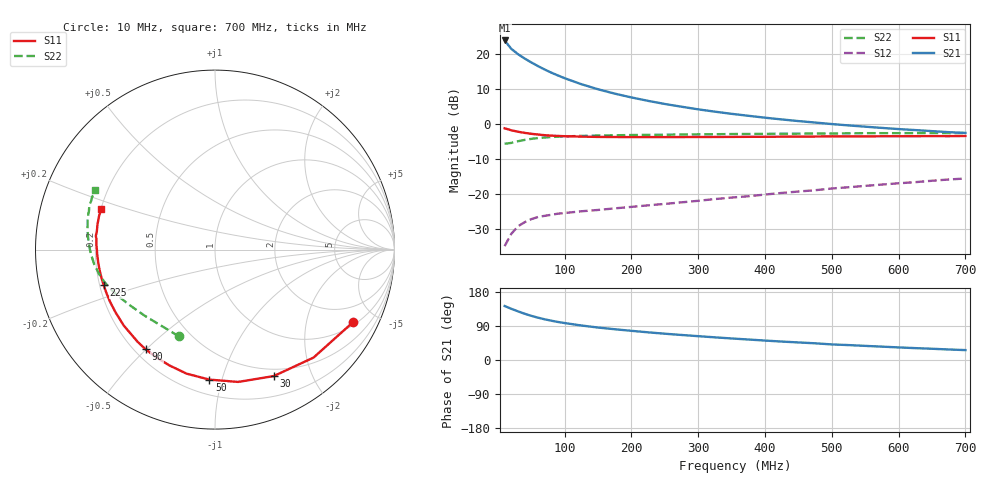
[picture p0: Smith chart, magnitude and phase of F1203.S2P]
! Date: Mon Aug 07 16:10:10 1995
# MHZ  S  MA  R  50.0000
!  POLYFET RF DEVICES
!  F1203
!  S PARAMETERS
!  VDS=12.5V, IDQ=200mA
! FREQ  S11MAG  S11ANG  S21MAG  S21ANG  S12MAG  S12ANG  S22MAG  S22ANG
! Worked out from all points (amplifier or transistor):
!   34 points, 10 MHz to 700 MHz, reference 50 ohm
!   highest |S21| = 23.8 dB at 10 MHz (marker M1)
!   |S21| within 3 dB of that: start of sweep to 24.06 MHz
!   unconditionally stable (mu >= 1): 188.4 MHz to end of sweep
!   at 60 MHz: K = 0.37, MSG = 21.5 dB, |S12| = -26.5 dB
!   at 300 MHz: K = 1.25, MAG = 10.0 dB, |S12| = -21.9 dB
!   at 700 MHz: K = 1.24, MAG = 3.5 dB, |S12| = -15.5 dB
!   S11 on the Smith chart (normalised r, x): 10 MHz: 1.14, -3.75; 30 MHz: 0.42, -1.49; 50 MHz: 0.30, -0.91; 90 MHz: 0.24, -0.50; 225 MHz: 0.22, -0.15; 700 MHz: 0.20, +0.17
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10  0.8697 -27.6  15.52 142.5  0.01819 56.1  0.5237 -112.5
20  0.8145 -47.6  11.79 135.1  0.02725 49.0  0.5383 -137.0
30  0.7771 -65.1  9.908 128.4  0.03489 44.9  0.5685 -147.3
40  0.7484 -80.1  8.584 122.1  0.03992 42.1  0.5939 -153.5
50  0.7251 -92.4  7.539 116.5  0.04413 39.8  0.6148 -157.9
60  0.7091 -102.8  6.689 111.7  0.0474 38.0  0.6308 -161.4
70  0.6935 -111.5  5.982 107.4  0.0492 35.8  0.6431 -164.0
80  0.6835 -118.7  5.391 103.7  0.05098 34.5  0.6521 -166.2
90  0.6769 -124.8  4.914 100.3  0.05283 34.7  0.6605 -168.1
100  0.6706 -130.0  4.495 97.5  0.054 34.0  0.6655 -169.8
125  0.6615 -140.3  3.693 91.1  0.05713 33.9  0.678 -173.1
150  0.6551 -147.9  3.127 85.6  0.0597 35.2  0.685 -175.8
175  0.653 -153.6  2.71 81.1  0.06287 36.2  0.6919 -178.1
200  0.6514 -158.4  2.392 77.0  0.06602 37.7  0.6971 179.9
225  0.6513 -162.2  2.137 73.0  0.06949 39.4  0.7008 178.3
250  0.6516 -165.6  1.93 69.3  0.0728 41.0  0.7044 176.6
300  0.6534 -171.2  1.618 62.9  0.0806 43.2  0.7133 173.5
375  0.6571 -177.9  1.311 54.1  0.09357 45.6  0.7215 169.5
425  0.6602 178.5  1.163 48.7  0.1043 46.4  0.7285 166.9
475  0.6634 174.8  1.05 44.1  0.1141 46.9  0.7336 164.3
600  0.67 166.6  0.8475 33.2  0.1432 45.4  0.7413 158.5
700  0.6756 160.4  0.7474 26.1  0.1674 42.9  0.7447 153.6
